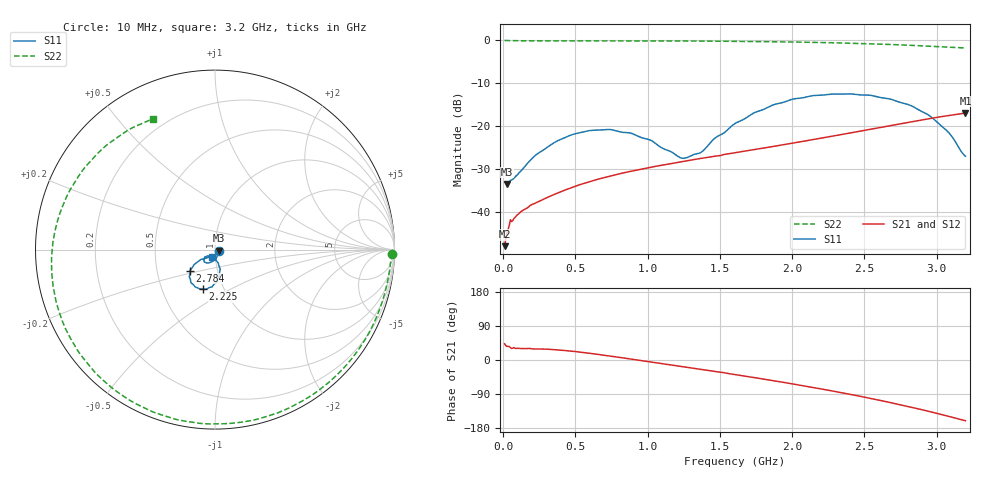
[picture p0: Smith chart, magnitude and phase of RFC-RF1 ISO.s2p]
!Agilent Technologies,N5230A,MY45001650,A.07.50.48
!Agilent N5230A: A.07.50.48
!Date: Monday, December 05, 2022 16:02:29
!Correction: S11(Full 2 Port(1,2))
!S21(Full 2 Port(1,2))
!S12(Full 2 Port(1,2))
!S22(Full 2 Port(1,2))
!S2P File: Measurements: S11, S21, S12, S22:
# Hz S  dB  R 50
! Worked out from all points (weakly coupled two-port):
!   400 points, 10 MHz to 3.2 GHz, reference 50 ohm
!   highest |S21| = -17.01 dB at 3.2 GHz (marker M1); lowest = -48.0 dB at 10 MHz (marker M2)
!   lowest |S11| = -33.5 dB at 25.99 MHz (marker M3), VSWR 1.04, Z = 52 - j0.682 ohm
!   |S11| at or under -10 dB: start of sweep to end of sweep
!   |S22| runs from -1.9 to -0.1 dB; largest |S21 - S12| = 0.00027
!   S11 on the Smith chart (normalised r, x): 10 MHz: 1.04, -0.01; 2.225 GHz: 0.80, -0.37; 2.784 GHz: 0.74, -0.18; 3.2 GHz: 0.96, -0.08
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1e7  -33.05 -16.2  -47.97 42.7  -48.16 43.9  -0.13 -1.3
2.598997e7  -33.53 -18.1  -44.97 35.9  -45.00 36.7  -0.13 -2.4
4.997494e7  -32.67 -24.8  -41.83 32.6  -42.07 33.0  -0.18 -4.7
5.796992e7  -32.60 -31.7  -42.26 30.5  -42.19 28.5  -0.18 -5.3
1.858897e8  -28.06 -71.8  -38.51 30.4  -38.53 30.5  -0.21 -16.3
3.617794e8  -23.73 -100.0  -35.83 27.2  -35.80 27.2  -0.22 -31.2
5.456642e8  -21.48 -118.2  -33.51 20.1  -33.51 20.1  -0.23 -46.5
7.295489e8  -20.83 -131.8  -31.76 11.0  -31.77 10.9  -0.23 -61.0
8.734586e8  -21.61 -140.0  -30.63 3.1  -30.63 3.1  -0.24 -71.9
1.081328e9  -24.76 -140.6  -29.24 -8.5  -29.25 -8.4  -0.25 -87.0
1.265213e9  -27.44 -114.4  -28.15 -18.9  -28.15 -18.9  -0.26 -99.6
1.377143e9  -25.98 -87.4  -27.52 -25.3  -27.52 -25.3  -0.28 -107.1
1.608997e9  -19.37 -75.1  -26.22 -38.6  -26.22 -38.6  -0.33 -122.1
1.864837e9  -15.17 -85.8  -24.81 -54.3  -24.81 -54.2  -0.42 -138.4
2.136667e9  -13.00 -101.5  -23.23 -71.9  -23.23 -71.8  -0.56 -155.9
2.224612e9  -12.79 -107.1  -22.70 -77.9  -22.70 -77.9  -0.62 -161.7
2.456466e9  -12.75 -121.1  -21.31 -94.6  -21.31 -94.6  -0.81 -177.8
2.672331e9  -13.70 -133.8  -19.99 -111.6  -19.99 -111.6  -1.05 165.7
2.784261e9  -14.84 -139.9  -19.30 -121.0  -19.30 -121.0  -1.20 156.4
2.97614e9  -18.28 -144.4  -18.16 -138.3  -18.16 -138.3  -1.49 138.7
3.08807e9  -21.70 -141.2  -17.55 -149.1  -17.55 -149.1  -1.68 127.4
3.2e9  -27.05 -114.9  -17.01 -160.2  -17.01 -160.2  -1.87 115.3
